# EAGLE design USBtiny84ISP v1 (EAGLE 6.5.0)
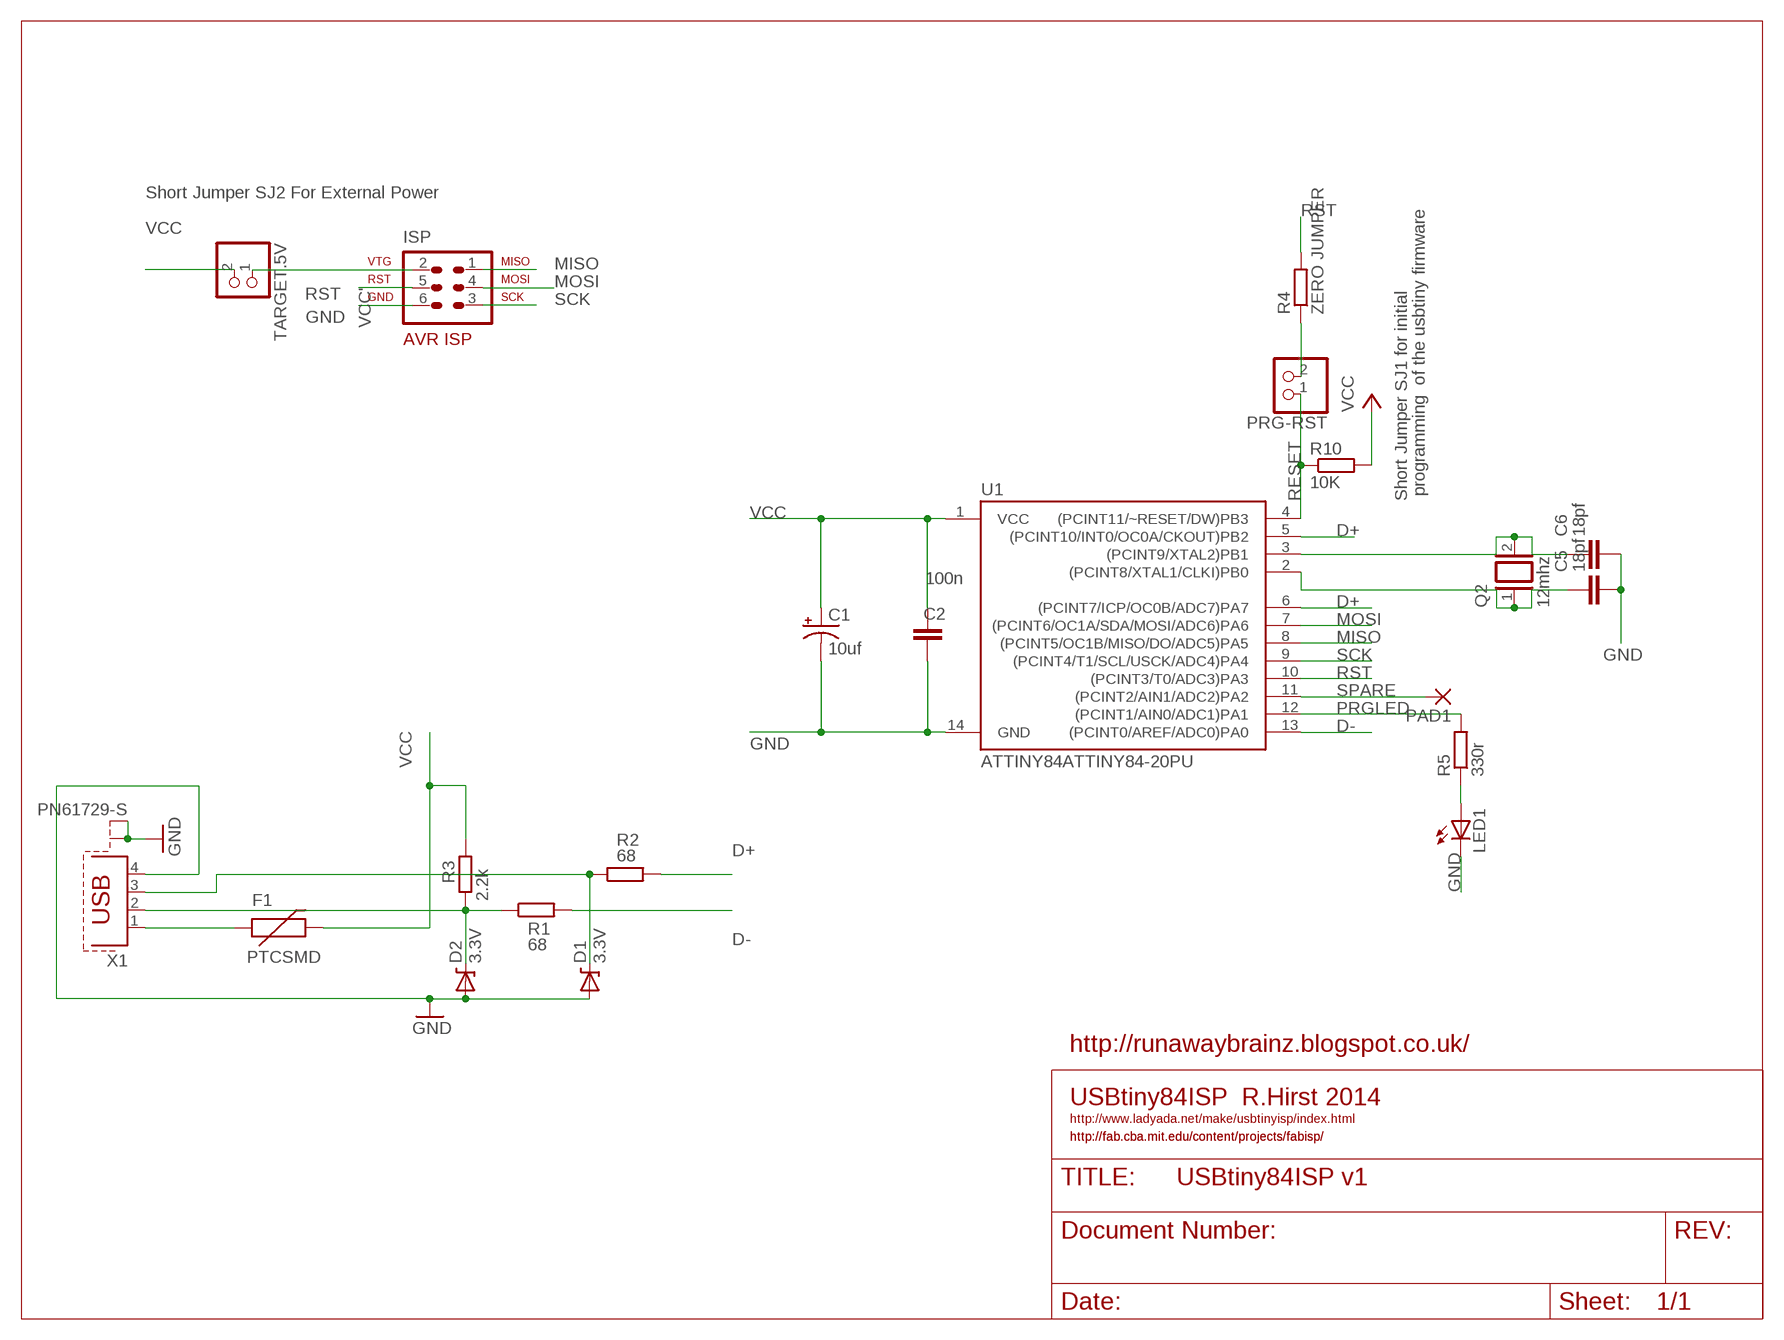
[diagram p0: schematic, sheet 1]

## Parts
C1  10uf  CPOL-USE2.5-6  [E2,5-6]
C2  100n  CAPACITOR_NPOL-PTH_0.1"  [C0.1PTH]
C5  18pf  CAPACITOR_NPOL-PTH_0.1"  [C0.1PTH]
C6  18pf  CAPACITOR_NPOL-PTH_0.1"  [C0.1PTH]
D1  3.3V  DIODE-ZENERPTH  [DIODE-ZENER]
D2  3.3V  DIODE-ZENERPTH  [DIODE-ZENER]
F1  PTCSMD  [PTC-1206]
ISP  AVR-ISP-6  [AVR-ISP-6]
LED1  LED3MM  [LED3MM]
PAD1  1,6/0,9  [1,6/0,9]
PRG-RST  PINHD-1X2  [1X02]
Q2  12mhz  XTAL/S  [QS]
R1  68  R-EU_0204/5  [0204/5]
R2  68  R-EU_0204/5  [0204/5]
R3  2.2k  R-EU_0204/5  [0204/5]
R4  ZERO JUMPER  R-EU_0204/5  [0204/5]
R5  330r  R-EU_0204/5  [0204/5]
R10  10K  R-EU_0204/5  [0204/5]
TARGET.5V  PINHD-1X2  [1X02]
U1  ATTINY84ATTINY84-20PU  [DIL14]
X1  PN61729-S  [PN61729-S]

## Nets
D+: R2.2 U1.5((PCINT10/INT0/OC0A/CKOUT)PB2) U1.6((PCINT7/ICP/OC0B/ADC7)PA7)
D-: R1.2 U1.13((PCINT0/AREF/ADC0)PA0)
DATA+: D1.P$1(C) R2.1 X1.3
DATA-: D2.P$1(C) R1.1 R3.1 X1.2
GND: C1.- C2.1 C5.2 C6.2 D1.P$2(A) D2.P$2(A) ISP.6 LED1.K(C) U1.14(GND) X1.4 X1.S1 X1.S2
MISO: ISP.1 U1.8((PCINT5/OC1B/MISO/DO/ADC5)PA5)
MOSI: ISP.4 U1.7((PCINT6/OC1A/SDA/MOSI/ADC6)PA6)
N$1: F1.1 X1.1
N$3: PRG-RST.2 R4.1
N$4: C5.1 Q2.1 U1.2((PCINT8/XTAL1/CLKI)PB0)
N$5: C6.1 Q2.2 U1.3((PCINT9/XTAL2)PB1)
N$8: LED1.A R5.1
PRGLED: R5.2 U1.12((PCINT1/AIN0/ADC1)PA1)
RESET: PRG-RST.1 R10.1 U1.4((PCINT11/~RESET/DW)PB3)
RST: ISP.5 R4.2 U1.10((PCINT3/T0/ADC3)PA3)
SCK: ISP.3 U1.9((PCINT4/T1/SCL/USCK/ADC4)PA4)
SPARE: PAD1.1(P) U1.11((PCINT2/AIN1/ADC2)PA2)
VCC: C1.+ C2.2 F1.2 R3.2 R10.2 TARGET.5V.2 U1.1(VCC)
VCC': ISP.2 TARGET.5V.1

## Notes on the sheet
- Short Jumper SJ2 For External Power
- Short Jumper SJ1 for initial | programming  of the usbtiny firmware
- http://runawaybrainz.blogspot.co.uk/
- USBtiny84ISP  R.Hirst 2014
- http://www.ladyada.net/make/usbtinyisp/index.html
- http://fab.cba.mit.edu/content/projects/fabisp/ | http://fab.cba.mit.edu/content/projects/fabisp/

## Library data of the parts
C1 = adafruit:CPOL-US: POLARIZED CAPACITOR, American symbol
C2 C5 C6 = dp_devices:CAPACITOR_NPOL: Non-Polarized capacitor in various packages
D1 D2 = SparkFun:DIODE-ZENER: Zener Diode
F1 = SparkFun:PTC: Resettable Fuse PTC
ISP = avr-4:AVR-ISP-6: AVR ISP-6 Serial Programming Header
LED1 = adafruit:LED: LED
PAD1 = wirepad:1,6/0,9: THROUGH-HOLE PAD
PRG-RST TARGET.5V = pinhead:PINHD-1X2: PIN HEADER
Q2 = special:XTAL/S: CRYSTAL
R1-R5 R10 = rcl:R-EU_: RESISTOR, European symbol
U1 = SparkFun-DigitalIC:ATTINY84: Atmel 14-pin 2/4/8kB flash uC
X1 = con-berg modified:PN61729-S: BERG USB connector; OC_FARNELL: unknown; OC_NEWARK: unknown

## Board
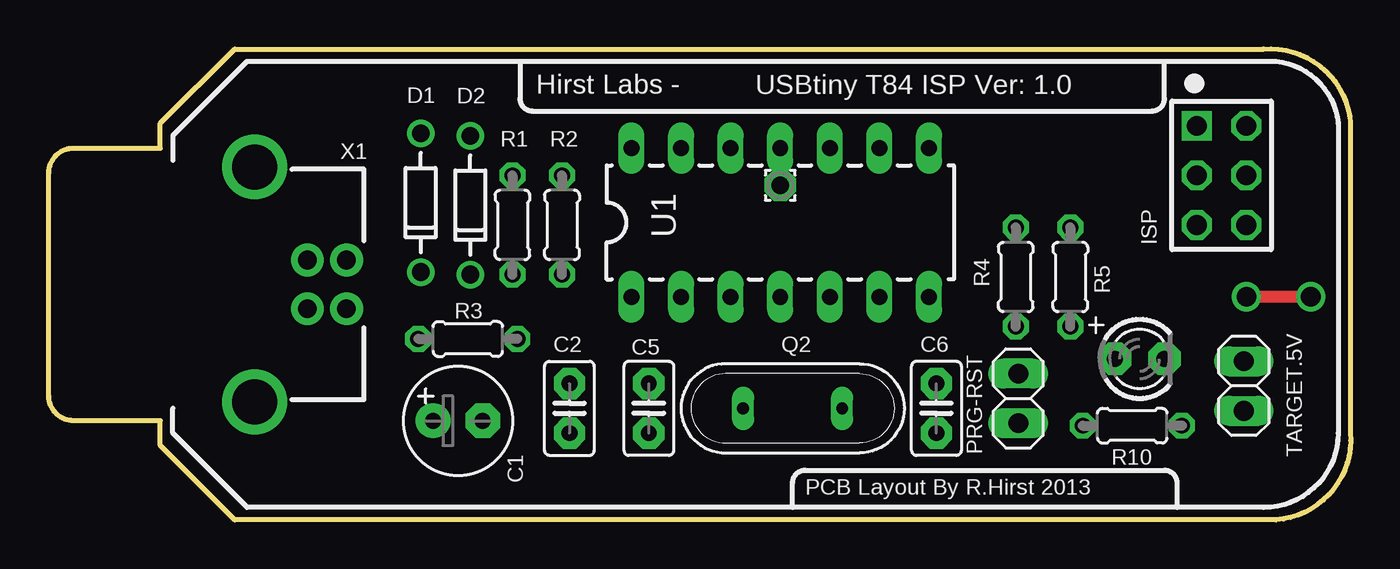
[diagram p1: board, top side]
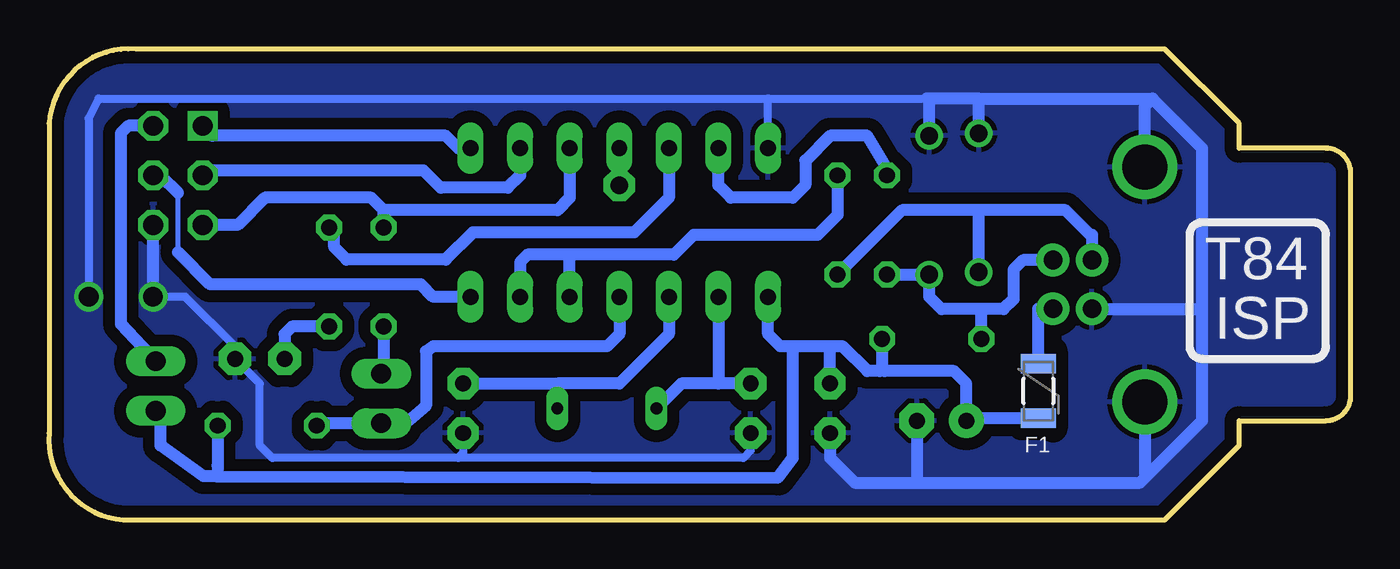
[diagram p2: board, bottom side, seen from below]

Size 66.69 x 24.14 mm. Coordinates in mm from the lower left corner, seen from the top.
Outline: 9.53,24.13 62.23,24.13 arc-90 66.67,20.32 66.67,4.44 arc-90 62.87,0 9.53,0 5.71,3.81 5.71,5.08 1.27,5.08 arc-90 0,6.35 0,17.78 arc-90 1.27,19.05 5.71,19.05 5.71,20.32 9.53,24.13
Copper layers (1*16): Top 0.035mm / dielectric 1.5mm / Bottom 0.035mm
Design rules "default *": minimum track width 12mil, minimum drill 24mil, track to track 17mil, track to pad 16mil, pad to pad 16mil, via to via 16mil, smd to smd 0mil, copper to edge 17mil, drill to drill 8mil, minimum pad ring 10mil, minimum via ring 8mil, stop-mask expansion 4mil, vias tented up to drill 0mil, thermal gap 10mil
bRestrict: 1 lines

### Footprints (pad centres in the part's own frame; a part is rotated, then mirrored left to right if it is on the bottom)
E2,5-6 = drill 0.813 pad 1.778: + -1.27,0 | drill 0.813 pad 1.778 octagon: - 1.27,0
C0.1PTH = drill 0.813 pad 1.6 octagon: 1 -1.27,0; 2 1.27,0
DIODE-ZENER = drill 0.9: P$1 -3.556,0; P$2 3.556,0
PTC-1206 = smd 1 x 1.8: 1 -1.4,0; 2 1.4,0
AVR-ISP-6 = drill 1.016 square: 1 -2.54,-1.27 | drill 1.016 octagon: 2 -2.54,1.27; 3 0,-1.27; 4 0,1.27; 5 2.54,-1.27; 6 2.54,1.27
LED3MM = drill 0.813 pad 1.676 octagon: A -1.27,0; K 1.27,0
1,6/0,9 = drill 0.914 pad 1.6 octagon: 1 0,0
1X02 = drill 1.016 long: 1 -1.27,0; 2 1.27,0
QS = drill 0.61 long: 1 -2.54,0; 2 2.54,0
0204/5 = drill 0.813 octagon: 1 -2.54,0; 2 2.54,0
DIL14 = drill 0.813 long: 1 -8.89,-3.81; 2 -6.35,-3.81; 3 -3.81,-3.81; 4 -1.27,-3.81; 5 1.27,-3.81; 6 3.81,-3.81; 7 6.35,-3.81; 8 6.35,3.81; 9 3.81,3.81; 10 1.27,3.81; 11 -1.27,3.81; 12 -3.81,3.81; 13 -6.35,3.81; 14 -8.89,3.81
PN61729-S = drill 0.95 pad 1.676: 1 1.25,4.71; 2 -1.25,4.71; 3 -1.25,2.71; 4 1.25,2.71 | drill 2.3 pad 2.9: S1 -6.02,0; S2 6.02,0

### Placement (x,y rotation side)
C1  20.96,5.08 0 top
C2  26.67,5.71 90 top
C5  30.73,5.71 270 top
C6  45.47,5.71 270 top
D1  19.05,16.26 90 top
D2  21.59,16.13 90 top
F1  16,6.6 270 bottom
ISP  60.07,17.65 270 top
LED1  55.88,8.26 0 top
PAD1  37.47,17.14 0 top
PRG-RST  49.66,6.22 90 top
Q2  38.1,5.71 0 top
R1  23.75,15.11 90 top
R2  26.29,15.11 90 top
R3  21.46,9.27 0 top
R4  49.53,12.45 90 top
R5  52.32,12.45 90 top
R10  55.5,4.83 0 top
TARGET.5V  61.21,6.86 270 top
U1  38.73,15.24 0 top
X1  10.54,12.07 270 top

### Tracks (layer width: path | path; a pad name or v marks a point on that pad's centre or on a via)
D+
  Bottom 0.61: R2.2 26.29,15.62 27.3,14.61 33.66,14.61 34.67,13.59 40.01,13.59 | 40.01,13.59 42.16,13.59 42.55,13.21 U1.6 | U1.5 40.01,13.59
D-
  Bottom 0.61: R1.2 23.75,18.03 24.77,19.68 26.67,19.68 27.94,18.41 27.94,17.14 28.57,16.51 31.75,16.51 32.38,17.14 U1.13
DATA+
  Bottom 0.61: 19.05,15.88 14.61,15.88 13.34,14.61 13.25,14.61 X1.3 | 19.05,15.88 22.99,15.88 R2.1 | D1.P$1 19.05,15.88
DATA-
  Bottom 0.61: R1.1 D2.P$1 | D2.P$1 21.59,12.45 | 19.05,10.79 17.78,10.79 17.27,11.3 17.27,12.83 16.78,13.32 X1.2 | 19.05,10.79 20.96,10.79 21.59,11.43 D2.P$1 | R3.1 18.92,10.67 19.05,10.79
GND  (via drill 1)
  Top 0.61: v64.64,11.43 v61.34,11.43
  Bottom 0.406: U1.14 29.84,21.59 | 29.84,21.59 21.72,21.59 21.59,21.59 | 29.84,21.59 64.14,21.59 64.64,20.57 v64.64,11.43 | C5.2 30.73,3.56 31.11,3.17 45.72,3.17 | 45.72,3.17 55.24,3.17 55.88,3.81 55.88,6.99 LED1.K 57.15,8.89 59.69,11.43 v61.34,11.43 | C6.2 45.47,3.43 45.72,3.17
  Bottom 0.61: v61.34,11.43 ISP.6 | C2.1 26.67,3.17 25.4,1.91 22.23,1.91 | 22.23,1.91 10.79,1.91 10.48,2.22 | 19.05,21.59 21.59,21.59 | C1.- 22.23,1.91 | D1.P$2 19.05,21.59 | D2.P$2 21.59,21.46 21.72,21.59 | 19.05,21.59 10.16,21.59 | 10.16,21.59 7.62,19.05 7.62,10.79 | 7.62,10.79 7.62,5.08 10.48,2.22 | X1.4 7.64,10.82 7.62,10.79 | X1.S1 10.54,21.21 10.16,21.59 | X1.S2 10.54,2.29 10.48,2.22
  pour Bottom (isolate 0.61): 66.67,24.13 66.67,-0.64 0,0 0,24.77
MISO
  Bottom 0.61: U1.8 45.72,19.05 46.35,19.68 58.29,19.68 ISP.1
MOSI
  Bottom 0.254: 60.07,13.72 60.07,16.76
  Bottom 0.406: ISP.4 60.96,17.65
  Bottom 0.61: 60.96,17.65 60.07,16.76 | U1.7 46.99,11.43 47.62,12.07 58.42,12.07 60.07,13.72
N$1
  Bottom 0.61: F1.1 16,10.82 X1.1
N$3
  Bottom 0.406: PRG-RST.2 49.53,8
  Bottom 0.61: R4.1 49.53,7.62 PRG-RST.2
N$4
  Bottom 0.61: C5.1 32.38,6.99 | 32.38,6.99 34.29,6.99 Q2.1 | U1.2 32.38,6.99
N$5
  Bottom 0.61: U1.3 34.93,9.53 37.47,6.99 40.64,6.99 | 40.64,6.99 Q2.2 | C6.1 40.64,6.99
N$8
  Bottom 0.61: R5.1 54.23,9.91 54.61,9.53 LED1.A
PRGLED
  Bottom 0.61: U1.12 34.93,16.51 36.7,14.73 44.96,14.73 46.35,13.34 51.44,13.34 52.07,13.97 52.07,14.73 R5.2
RESET
  Bottom 0.61: U1.4 37.47,9.53 38.1,8.89 46.99,8.89 47.37,8.64 47.37,5.84 48.26,5.08 49.53,5.08 PRG-RST.1 52.83,4.95 R10.1
RST
  Bottom 0.61: U1.10 40.01,16.51 40.64,15.88 49.53,15.88 | ISP.5 57.02,15.11 55.63,16.51 50.16,16.51 49.53,15.88 | R4.2 49.53,15.88
SCK
  Bottom 0.61: U1.9 42.55,17.65 43.18,17.02 46.61,17.02 47.5,17.91 58.55,17.91 ISP.3
SPARE
  Bottom 0.61: U1.11 PAD1.1
VCC
  Bottom 0.61: 26.67,8.89 26.04,8.89 24.77,7.62 24.13,7.62 24,7.75 | 26.67,8.89 28.57,8.89 | 28.57,8.89 29.21,8.89 29.84,9.53 U1.1 | R3.2 24,7.75 | C2.2 26.67,8.89 | 58.07,2.22 29.34,2.16 28.57,3.17 28.57,8.89 | R10.2 58.05,2.78 58.07,2.22 | F1.2 19.56,5.2 C1.+ 19.68,6.99 20.32,7.62 23.88,7.62 24,7.75 | 58.07,2.22 58.76,2.23 60.96,3.81 60.96,5.33 TARGET.5V.2
VCC'
  Bottom 0.61: ISP.2 62.61,20.19 62.99,19.81 62.99,10.03 TARGET.5V.1

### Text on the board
_tsilk: Hirst Labs - | USBtiny T84 ISP Ver: 1.0 | PCB Layout By R.Hirst 2013
_bsilk: T84 | ISP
